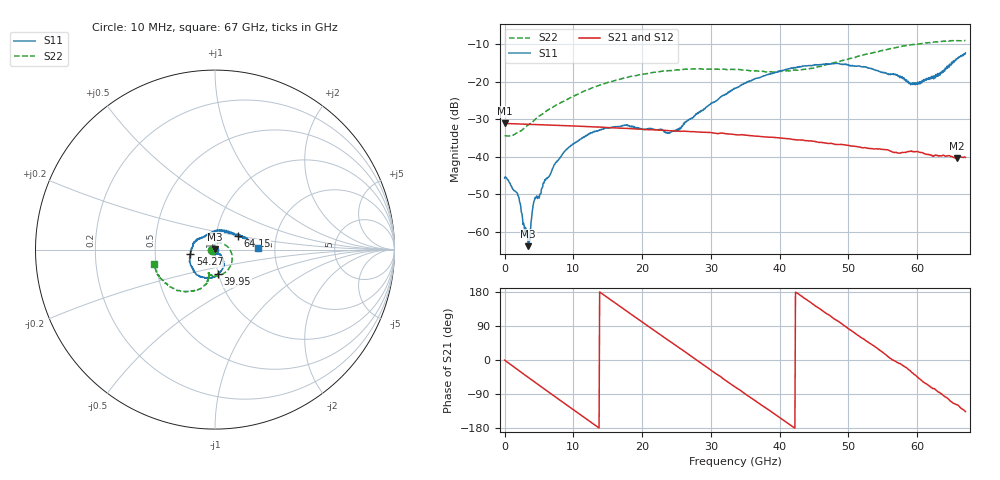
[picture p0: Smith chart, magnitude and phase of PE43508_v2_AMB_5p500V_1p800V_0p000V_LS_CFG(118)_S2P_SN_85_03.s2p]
!Keysight Technologies,N5227A,US51270237,A.10.43.00
!Date: Wednesday, August 22, 2018 17:19:01
!Correction: S11(Full 2 Port(1,3))
!S31(Full 2 Port(1,3))
!S13(Full 2 Port(1,3))
!S33(Full 2 Port(1,3))
!S2P File: Measurements: S11, S31, S13, S33:
# Hz S  dB  R 50
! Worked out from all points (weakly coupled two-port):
!   801 points, 10 MHz to 67 GHz, reference 50 ohm
!   highest |S21| = -31.14 dB at 10 MHz (marker M1); lowest = -40.4 dB at 65.74 GHz (marker M2)
!   lowest |S11| = -63.8 dB at 3.443 GHz (marker M3), VSWR 1.00, Z = 50 + j0.0582 ohm
!   |S11| at or under -10 dB: start of sweep to end of sweep
!   |S22| runs from -34.5 to -9.1 dB; largest |S21 - S12| = 0.00015
!   S11 on the Smith chart (normalised r, x): 10 MHz: 0.99, -0.00; 39.95 GHz: 1.00, -0.28; 54.27 GHz: 0.76, -0.04; 64.15 GHz: 1.27, +0.19; 67 GHz: 1.63, +0.03
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1e7  -45.67 -176.5  -31.14 -0.2  -31.13 -0.3  -34.47 -179.8
1.935962e9  -50.23 155.9  -31.27 -26.1  -31.27 -26.1  -33.50 129.4
2.857075e9  -58.49 117.9  -31.33 -38.2  -31.33 -38.3  -32.42 108.8
3.443238e9  -63.79 64.2  -31.37 -45.9  -31.37 -46.0  -31.60 98.3
3.69445e9  -62.06 4.9  -31.39 -49.2  -31.39 -49.3  -31.29 94.0
4.36435e9  -51.45 -2.6  -31.42 -57.9  -31.43 -58.0  -30.24 83.2
5.787888e9  -46.64 -23.9  -31.51 -76.5  -31.52 -76.5  -28.27 65.7
8.7187e9  -38.58 -54.4  -31.73 -114.5  -31.72 -114.6  -25.16 35.4
1.123082e10  -35.01 -64.7  -31.92 -147.0  -31.92 -147.0  -22.86 12.5
1.74274e10  -31.68 -88.1  -32.44 133.4  -32.44 133.4  -19.05 -31.1
2.236791e10  -32.76 -84.5  -32.92 70.3  -32.92 70.3  -17.43 -59.0
2.513125e10  -32.65 -65.4  -33.19 35.5  -33.19 35.4  -16.86 -71.8
3.3505e10  -21.85 -55.3  -34.10 -71.2  -34.11 -71.2  -16.79 -99.9
3.995279e10  -17.17 -82.7  -35.00 -151.5  -34.98 -151.4  -17.26 -105.4
4.472582e10  -15.72 -106.9  -35.84 148.7  -35.84 148.8  -16.49 -102.4
4.841028e10  -15.17 -127.0  -36.76 103.3  -36.75 103.2  -14.83 -103.2
5.42719e10  -17.17 -170.4  -37.92 29.6  -37.89 29.4  -12.06 -115.5
5.586291e10  -18.19 171.3  -38.30 6.8  -38.30 6.6  -11.34 -120.6
5.979858e10  -20.36 113.1  -38.62 -40.7  -38.60 -41.1  -10.13 -134.7
6.415292e10  -16.67 30.2  -39.90 -97.8  -39.96 -98.2  -9.27 -153.3
6.574394e10  -14.11 13.7  -40.38 -118.7  -40.41 -119.0  -9.14 -160.4
6.7e10  -12.38 1.8  -40.18 -136.1  -40.27 -136.2  -9.09 -167.0
